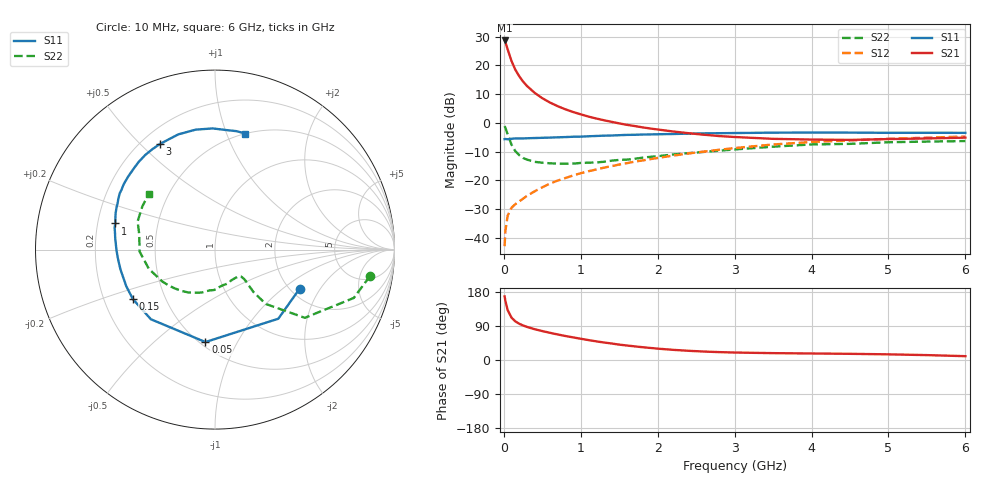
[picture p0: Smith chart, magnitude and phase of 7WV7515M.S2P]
! Infineon Technologies  Discrete & RF Semiconductors
! BFS17W
! Si NPN RF Bipolar Junction Transistor in SOT323
! VCE = 0.75 V  IC = 15 mA
! Common Emitter S-Parameters:  August  1999
# GHz  S  MA  R  50
!  f  S11  S21  S12  S22
! GHz  MAG  ANG  MAG  ANG  MAG  ANG  MAG  ANG
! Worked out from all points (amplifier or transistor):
!   36 points, 10 MHz to 6 GHz, reference 50 ohm
!   highest |S21| = 28.7 dB at 10 MHz (marker M1)
!   |S21| within 3 dB of that: start of sweep to 48.39 MHz
!   unconditionally stable (mu >= 1): 151.8 MHz to end of sweep
!   at 250 MHz: K = 1.34, MAG = 16.9 dB, |S12| = -26.4 dB
!   at 1.4 GHz: K = 1.65, MAG = 3.0 dB, |S12| = -15.1 dB
!   at 6 GHz: K = 1.14, MAG = -2.5 dB, |S12| = -4.8 dB
!   S11 on the Smith chart (normalised r, x): 10 MHz: 2.23, -1.33; 50 MHz: 0.53, -0.75; 150 MHz: 0.32, -0.25; 1 GHz: 0.27, +0.12; 3 GHz: 0.27, +0.57; 6 GHz: 0.50, +1.17
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0.01  0.5193 -24.9  27.21 167.8  0.0071 76.6  0.876 -9.7
0.02  0.5222 -47.5  25.5 156.0  0.013 73.1  0.8189 -19.2
0.05  0.5178 -95.9  18.96 131.4  0.0243 54.6  0.6285 -37.2
0.1  0.5274 -132.6  11.88 111.7  0.0332 46.0  0.4152 -46.9
0.15  0.5343 -148.9  8.392 101.8  0.0383 46.6  0.3201 -47.8
0.2  0.5348 -157.7  6.474 95.7  0.0427 49.6  0.2738 -46.7
0.25  0.5348 -164.0  5.234 91.1  0.0477 51.4  0.2448 -45.6
0.3  0.5383 -168.3  4.395 87.4  0.0534 54.6  0.2288 -45.3
0.4  0.5432 -174.8  3.334 81.3  0.064 57.8  0.2092 -45.9
0.5  0.5483 -179.3  2.684 76.3  0.0754 60.0  0.202 -47.4
0.6  0.5528 177.2  2.252 71.7  0.0874 61.2  0.1971 -50.1
0.8  0.5645 170.7  1.719 63.3  0.1092 62.7  0.1935 -58.8
1  0.5747 165.3  1.405 56.1  0.1326 63.1  0.1999 -66.8
1.1  0.583 162.1  1.285 52.5  0.1435 62.8  0.2021 -72.7
1.3  0.5972 156.6  1.109 46.2  0.1655 62.3  0.2096 -83.1
1.6  0.6163 149.5  0.922 38.2  0.1982 61.4  0.2285 -97.1
2.2  0.6387 135.5  0.706 26.8  0.2684 58.0  0.2804 -121.4
3  0.6637 117.6  0.566 19.7  0.3635 50.3  0.3434 -148.8
3.5  0.6738 107.7  0.526 18.1  0.4193 44.3  0.3839 -163.8
4.5  0.6753 91.1  0.504 16.3  0.4921 31.8  0.4299 168.9
5.5  0.6707 79.6  0.534 12.9  0.5512 21.7  0.4711 149.3
6  0.6683 75.3  0.552 10.1  0.5773 16.9  0.4811 140.3
